TYPE ST_Status_UDINT_TO_BIT :
STRUCT
	Latch_C_valid					:	BIT;
	Latch_extern_valid				:	BIT;
	Set_counter_done				:	BIT;
	Counter_underflow				:	BIT;
	Counter_overflow				:	BIT;
	Status_of_input_status			:	BIT;
	Open_circuit					:	BIT;
	Extrapolation_stall				:	BIT;
	
	Status_of_input_A				:	BIT;
	Status_of_input_B				:	BIT;
	Status_of_input_C				:	BIT;
	Status_of_input_gate			:	BIT;
	Diag							:	BIT;
	TxPDO_State						:	BIT;
	Input_cycle_counter_L_BIT		:	BIT;// ST_BIT2 不行，会自动补齐
	Input_cycle_counter_H_BIT		:	BIT;
	
	Software_gate_valid				:	BIT;
	Latch_extern_2_valid			:	BIT;
	Direction_inversion_detected	:	BIT;
	Status_of_extern_latch			:	BIT;
	Counter_value_out_of_range		:	BIT;
	{attribute 'hide'}
	reserve_b22						:	BIT;
	{attribute 'hide'}
	reserve_b23						:	BIT;
	{attribute 'hide'}
	reserve_b24						:	BIT;
	{attribute 'hide'}
	reserve_byte					:	USINT;
END_STRUCT
END_TYPE
